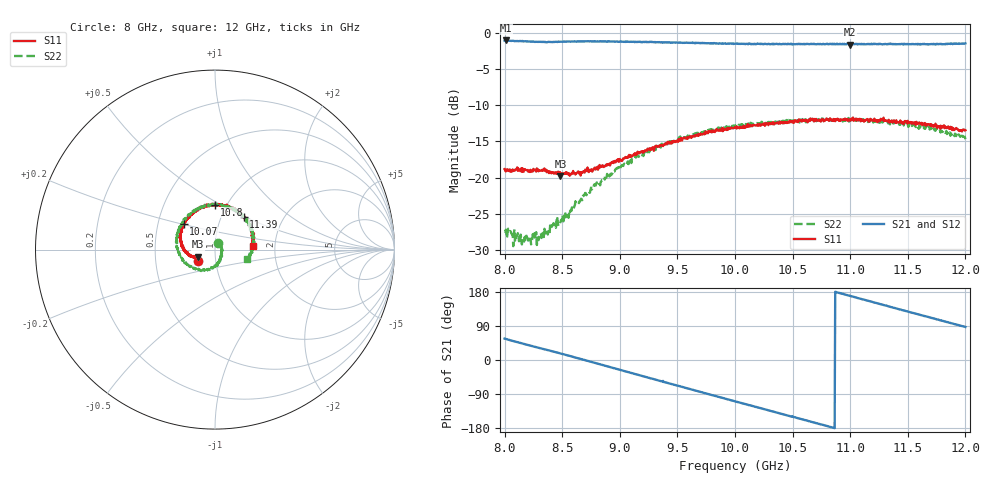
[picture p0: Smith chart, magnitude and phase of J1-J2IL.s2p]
!Agilent Technologies,N5230C,MY49001174,A.09.42.21
!Agilent N5230C: A.09.42.21
!Date: Saturday, January 30, 2016 08:42:10
!Correction: S11(Full 2 Port(1,2))
!S21(Full 2 Port(1,2))
!S12(Full 2 Port(1,2))
!S22(Full 2 Port(1,2))
!S2P File: Measurements: S11, S21, S12, S22:
# Hz S  dB  R 50
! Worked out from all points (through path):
!   801 points, 8 GHz to 12 GHz, reference 50 ohm
!   highest |S21| = -1.09 dB at 8.015 GHz (marker M1); lowest = -1.7 dB at 10.99 GHz (marker M2)
!   group delay of S21, straight-line fit = 229 ps
!   lowest |S11| = -19.8 dB at 8.485 GHz (marker M3), VSWR 1.23, Z = 41.2 - j3.26 ohm
!   |S11| at or under -10 dB: start of sweep to end of sweep
!   |S22| runs from -29.5 to -11.8 dB; largest |S21 - S12| = 0.014
!   S11 on the Smith chart (normalised r, x): 8 GHz: 0.82, -0.10; 10.07 GHz: 0.68, +0.20; 10.8 GHz: 0.88, +0.47; 11.39 GHz: 1.27, +0.49; 12 GHz: 1.53, +0.07
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8e9  -18.83 -146.9  -1.14 56.4  -1.10 56.3  -27.46 66.8
8.015e9  -18.91 -146.0  -1.09 55.2  -1.11 55.1  -27.45 63.8
8.22e9  -19.23 -152.3  -1.23 38.1  -1.27 38.1  -28.56 8.4
8.3e9  -19.01 -155.3  -1.27 31.7  -1.33 31.9  -28.17 -16.2
8.485e9  -19.79 -157.6  -1.28 17.3  -1.28 17.4  -26.11 -47.9
8.67e9  -19.34 -158.6  -1.22 1.9  -1.21 1.9  -23.04 -71.8
8.825e9  -18.26 -158.9  -1.22 -10.9  -1.21 -11.0  -20.89 -90.3
8.98e9  -17.66 -162.3  -1.25 -24.2  -1.24 -24.2  -18.72 -109.1
9.335e9  -15.73 -176.7  -1.35 -54.0  -1.33 -53.8  -15.65 -142.5
9.54e9  -14.89 174.2  -1.41 -71.0  -1.36 -70.9  -14.30 -162.7
9.685e9  -14.22 165.3  -1.43 -83.1  -1.42 -83.0  -13.92 -175.3
1e10  -13.05 146.1  -1.55 -109.1  -1.55 -109.1  -12.83 156.4
1.007e10  -12.95 141.2  -1.55 -114.6  -1.59 -114.9  -12.83 150.6
1.039e10  -12.29 120.5  -1.58 -140.8  -1.55 -141.0  -12.39 123.3
1.067e10  -12.06 102.8  -1.57 -163.9  -1.61 -163.4  -11.89 100.3
1.0805e10  -12.03 90.5  -1.59 -174.4  -1.57 -174.9  -12.07 89.4
1.0995e10  -12.01 77.5  -1.66 169.4  -1.52 169.4  -12.00 74.1
1.1165e10  -12.28 65.6  -1.61 155.4  -1.57 155.8  -12.12 58.2
1.1335e10  -12.03 53.9  -1.59 141.5  -1.61 141.4  -12.39 42.6
1.139e10  -12.31 49.0  -1.60 137.0  -1.61 136.8  -12.37 38.7
1.1675e10  -12.73 26.3  -1.63 113.8  -1.55 113.9  -13.14 11.7
1.2e10  -13.48 6.0  -1.49 87.2  -1.52 87.1  -14.70 -16.4
